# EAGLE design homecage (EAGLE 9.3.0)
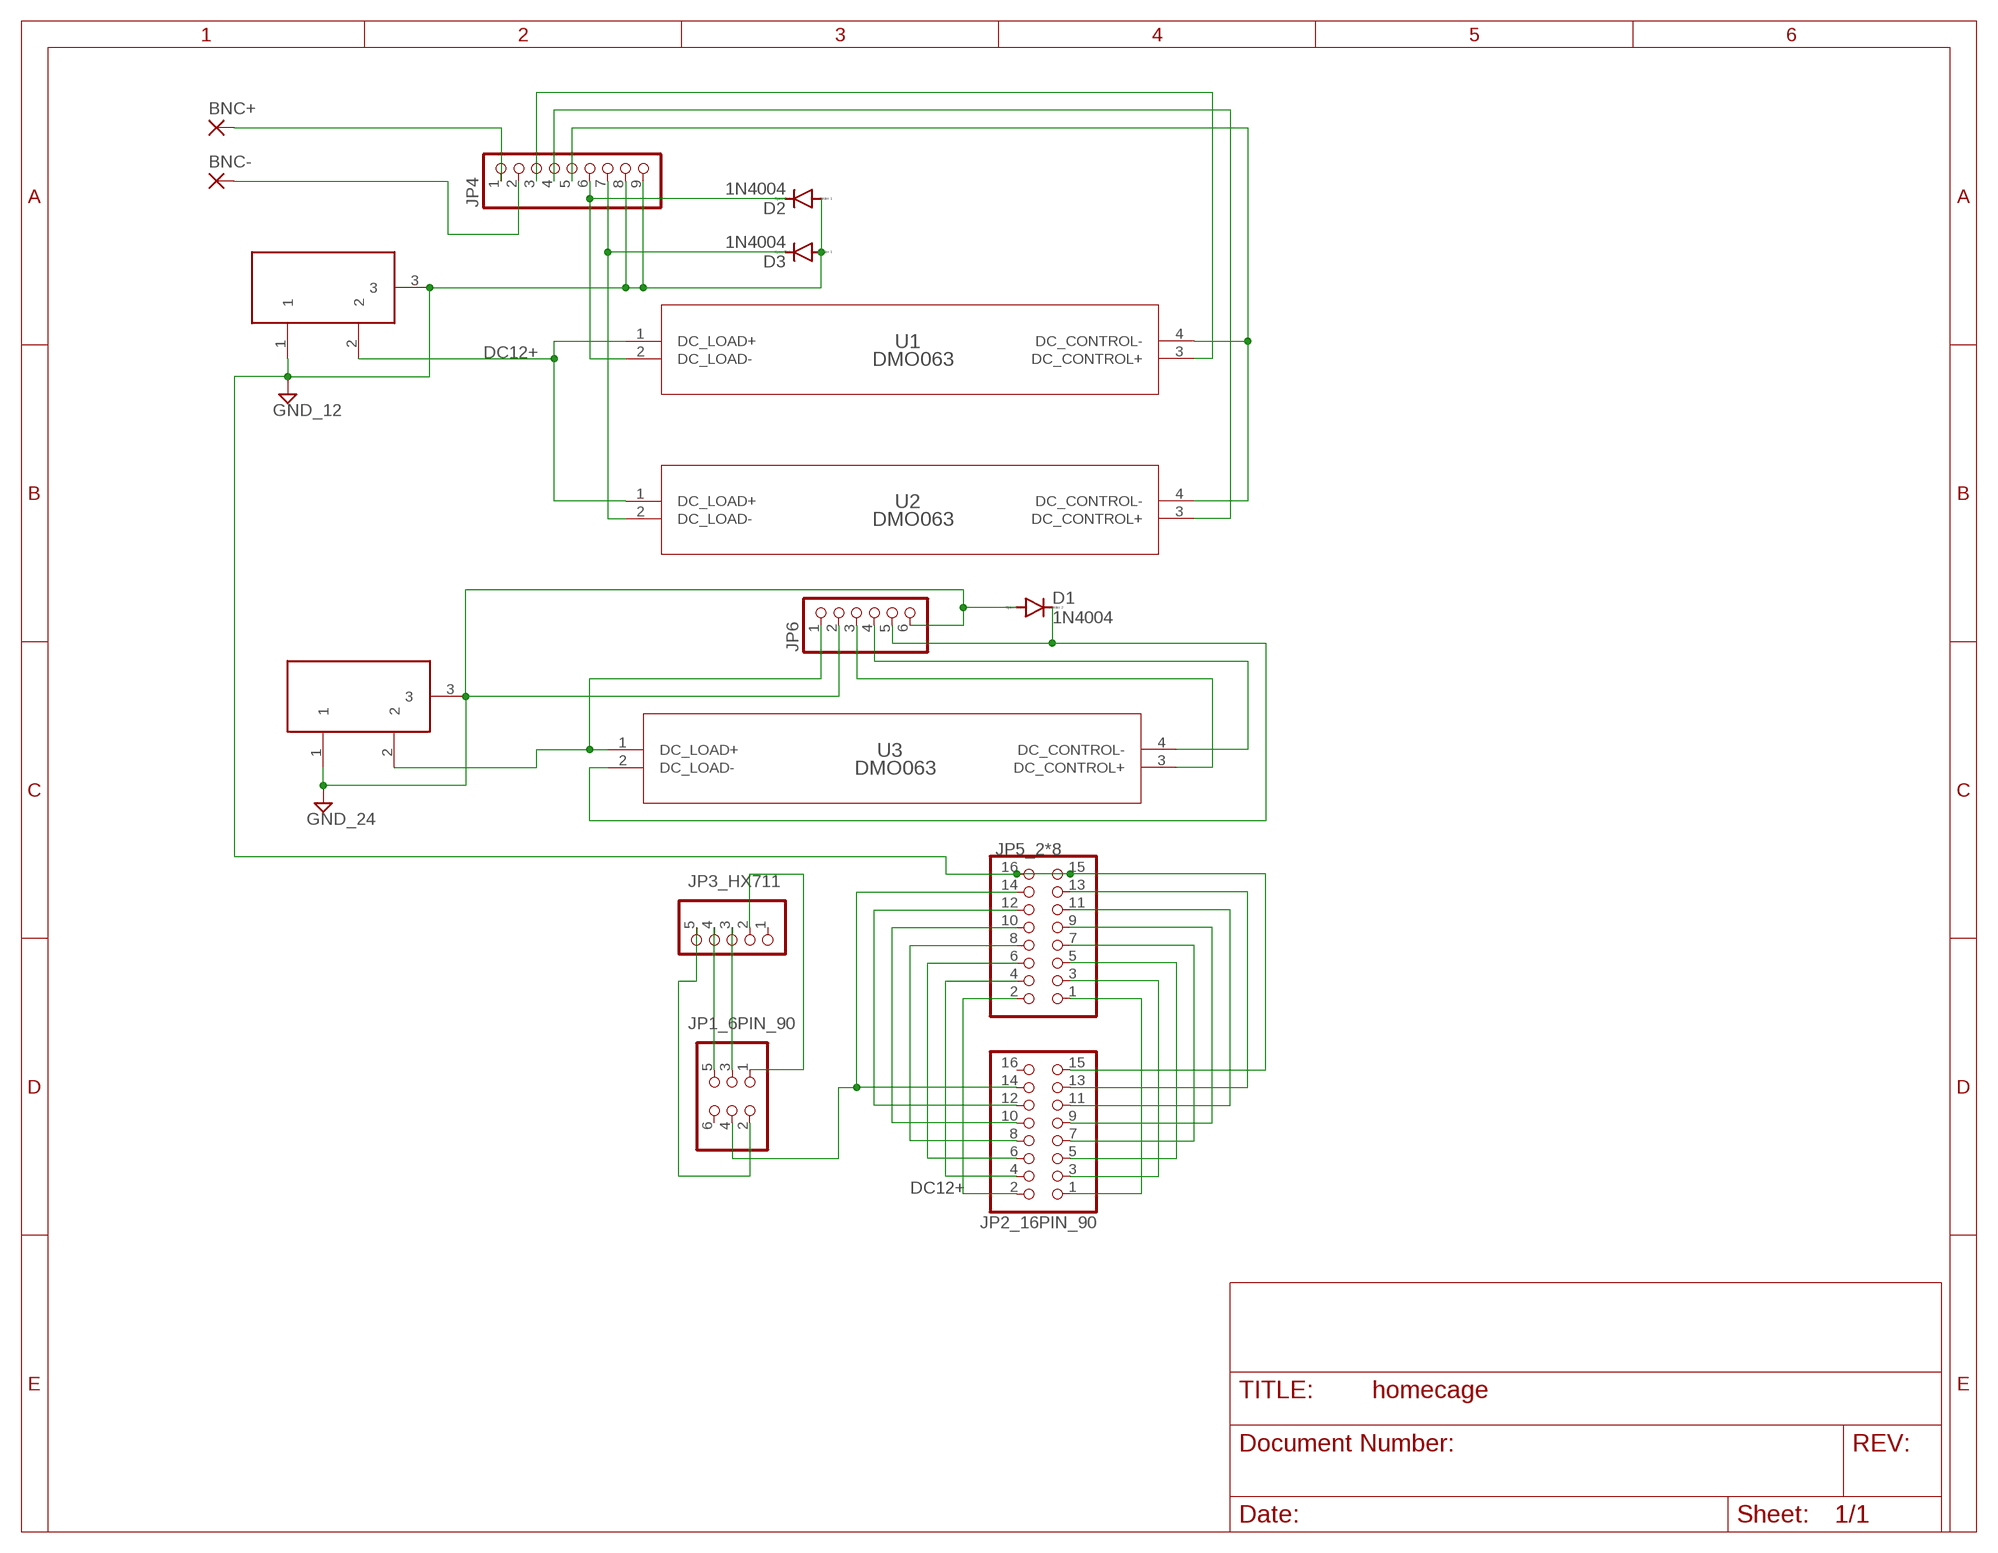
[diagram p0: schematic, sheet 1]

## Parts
BNC+  SMD5  [SMD2,54-5,08]
BNC-  SMD5  [SMD2,54-5,08]
D1  1N4004  [DO41-10]
D2  1N4004  [DO41-10]
D3  1N4004  [DO41-10]
DC12V  POWERSUPPLY_DC21MMX  [POWERSUPPLY_DC-21MM]
DC24V  POWERSUPPLY_DC21MMX  [POWERSUPPLY_DC-21MM]
JP1_6PIN_90  PINHD-2X3/90  [2X03/90]
JP2_16PIN_90  PINHD-2X8/90  [2X08/90]
JP3_HX711  PINHD-1X5  [1X05]
JP4  PINHD-1X9  [1X09]
JP5_2*8  PINHD-2X8  [2X08]
JP6  PINHD-1X6  [1X06]
U1  DMO063  [SIP-4_DMO]
U2  DMO063  [SIP-4_DMO]
U3  DMO063  [SIP-4_DMO]

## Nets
DC12+ [power]: DC12V.2 JP2_16PIN_90.2 JP5_2*8.2 U1.1(DC_LOAD+) U2.1(DC_LOAD+)
GND1 [power]: D2.A D3.A DC12V.1 DC12V.3 JP2_16PIN_90.15 JP4.8 JP4.9 JP5_2*8.15 JP5_2*8.16 ; supply symbol labelled GND_12
GND2 [power]: D1.A DC24V.1 DC24V.3 JP6.2 JP6.6 ; supply symbol labelled GND_24
N$1: JP2_16PIN_90.1 JP5_2*8.1
N$2: JP2_16PIN_90.3 JP5_2*8.3
N$3: JP2_16PIN_90.5 JP5_2*8.5
N$4: JP2_16PIN_90.7 JP5_2*8.7
N$5: JP2_16PIN_90.9 JP5_2*8.9
N$6: JP2_16PIN_90.11 JP5_2*8.11
N$7: JP2_16PIN_90.13 JP5_2*8.13
N$8: D2.C JP4.6 U1.2(DC_LOAD-)
N$10: JP2_16PIN_90.4 JP5_2*8.4
N$11: JP2_16PIN_90.6 JP5_2*8.6
N$12: JP2_16PIN_90.8 JP5_2*8.8
N$13: JP2_16PIN_90.10 JP5_2*8.10
N$14: JP2_16PIN_90.12 JP5_2*8.12
N$15: JP1_6PIN_90.4 JP2_16PIN_90.14 JP5_2*8.14
N$17: JP1_6PIN_90.1 JP3_HX711.2
N$18: JP1_6PIN_90.3 JP3_HX711.3
N$19: JP1_6PIN_90.5 JP3_HX711.4
N$20: JP1_6PIN_90.2 JP3_HX711.5
N$22 [power]: DC24V.2 JP6.1 U3.1(DC_LOAD+)
N$23: D3.C JP4.7 U2.2(DC_LOAD-)
N$24: JP4.5 U1.4(DC_CONTROL-) U2.4(DC_CONTROL-)
N$25: BNC+.1(P) JP4.1
N$26: JP4.4 U2.3(DC_CONTROL+)
N$27: JP4.3 U1.3(DC_CONTROL+)
N$28: BNC-.1(P) JP4.2
N$30: JP6.3 U3.3(DC_CONTROL+)
N$31: JP6.4 U3.4(DC_CONTROL-)
N$32: D1.C JP6.5 U3.2(DC_LOAD-)
Unconnected: JP1_6PIN_90.6 JP2_16PIN_90.16 JP3_HX711.1

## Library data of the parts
BNC+ BNC- = wirepad:SMD5: SMD PAD
D1-D3 = diode:1N4004: DIODE
DC12V DC24V = Arduino_MEGA2560_ref:POWERSUPPLY_DC21MM
JP1_6PIN_90 = pinhead:PINHD-2X3: PIN HEADER
JP2_16PIN_90 JP5_2*8 = pinhead:PINHD-2X8: PIN HEADER
JP3_HX711 = pinhead:PINHD-1X5: PIN HEADER
JP4 = pinhead:PINHD-1X9: PIN HEADER
JP6 = pinhead:PINHD-1X6: PIN HEADER
U1-U3 = homecage:DMO063; MANUFACTURER_PART_NUMBER: DMO063; VENDOR: Crydom

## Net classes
0 default: width 0.406 mm
1 power: width 1.219 mm

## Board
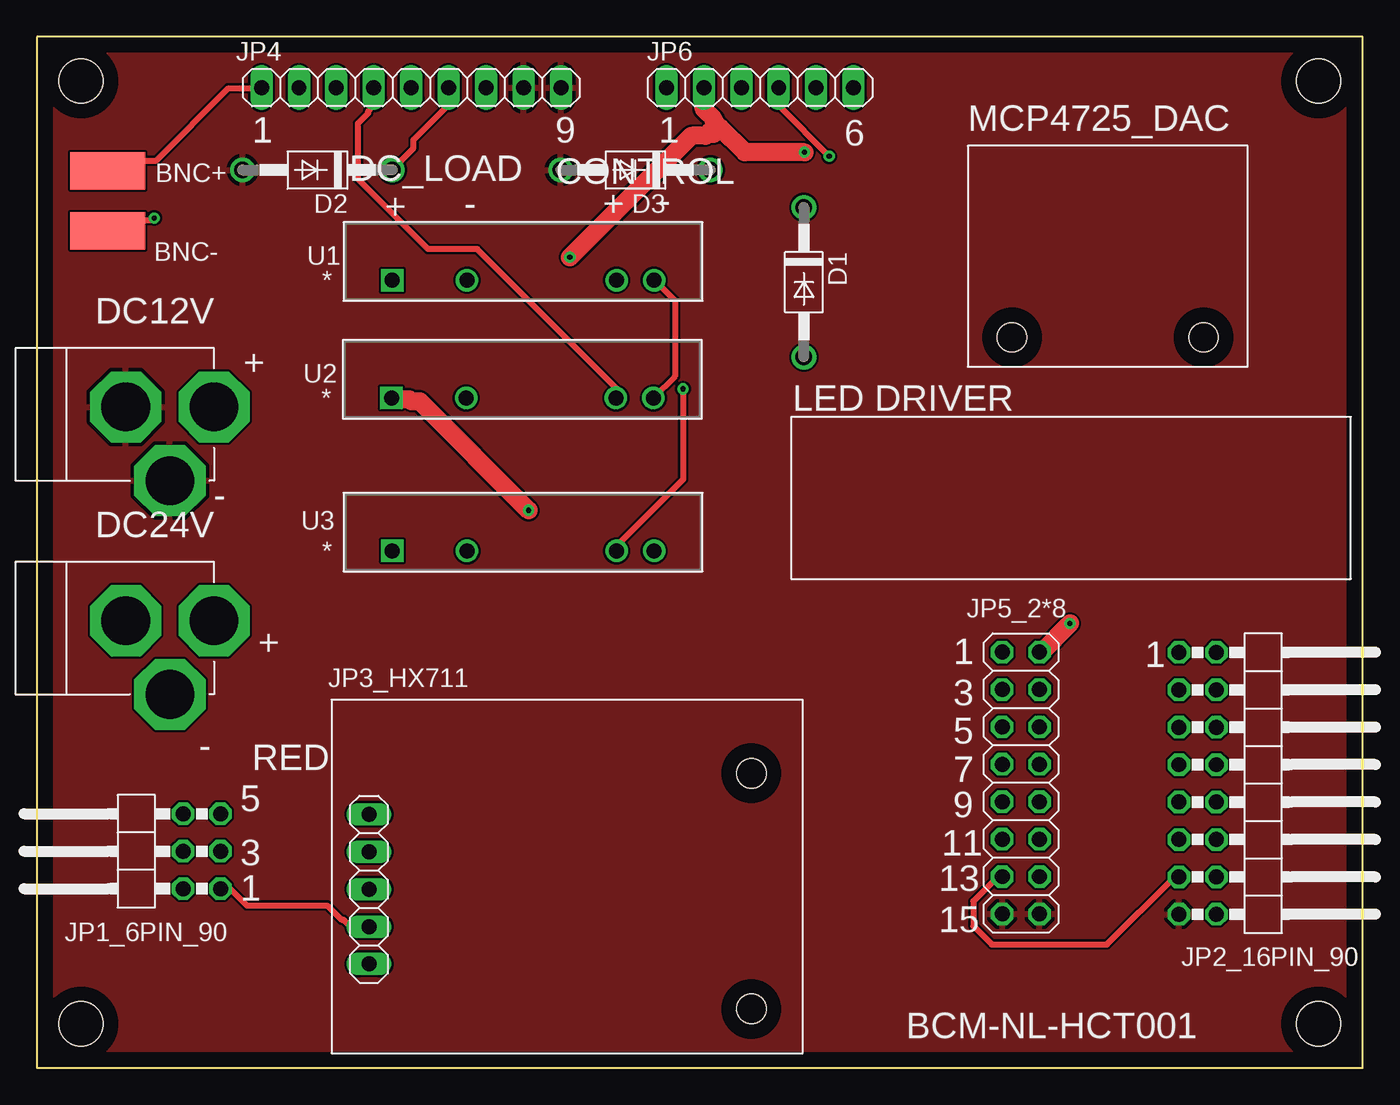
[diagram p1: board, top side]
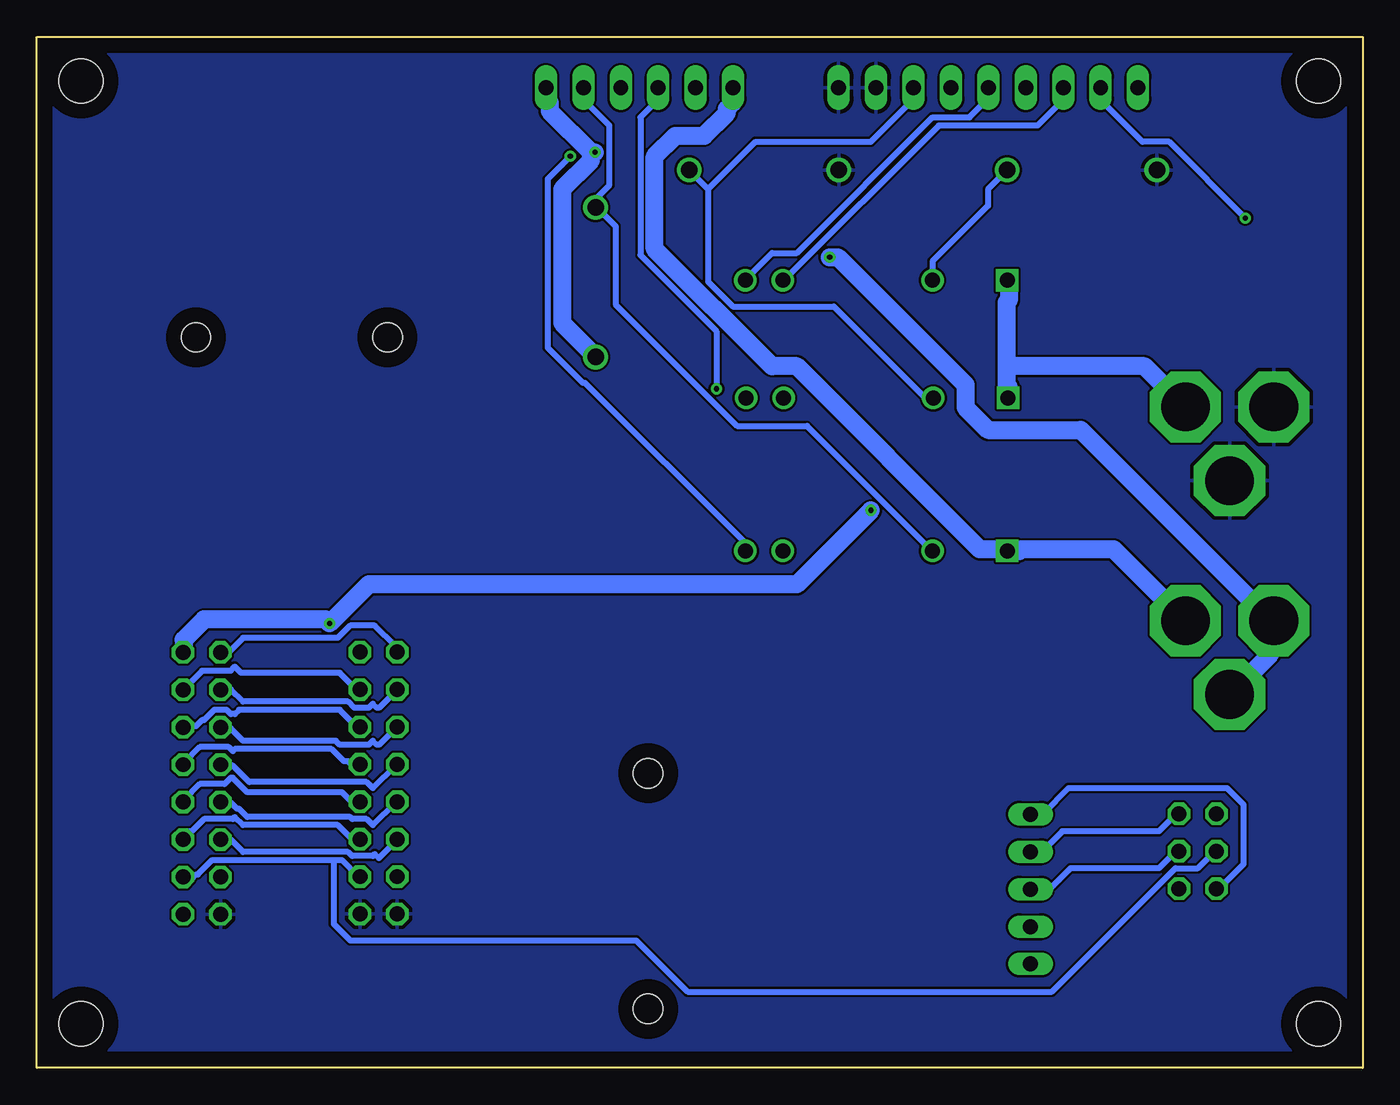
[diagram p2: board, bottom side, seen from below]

Size 90 x 70 mm. Coordinates in mm from the lower left corner, seen from the top.
Outline: 0,0 90,0 90,70 0,70 0,0
Copper layers (1*16): Top 0.035mm / dielectric 1.5mm / Bottom 0.035mm
Design rules "default": minimum track width 6mil, minimum drill 0.35mm, track to track 6mil, track to pad 6mil, pad to pad 6mil, via to via 6mil, smd to smd 6mil, copper to edge 40mil, drill to drill 6mil, minimum pad ring 10mil, minimum via ring 8mil, stop-mask expansion 4mil, vias tented up to drill 0mil, thermal gap 10mil
Holes 3 mm at 3,3 3,67 87,67 87,3
Holes 2 mm at 48.5,20 48.5,4 66.2,49.6 79.2,49.6

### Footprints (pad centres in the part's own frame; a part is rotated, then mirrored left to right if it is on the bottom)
SMD2,54-5,08 = smd 2.54 x 5.08: 1 0,0
DO41-10 = drill 1.118: A 5.08,0; C -5.08,0
POWERSUPPLY_DC-21MM = drill 3.302 pad 4.826 octagon: 1 -5.08,-3.353; 2 -0.076,-6.35; 3 -0.076,-0.356
2X03/90 = drill 1.016 octagon: 1 -2.54,-6.35; 2 -2.54,-3.81; 3 0,-6.35; 4 0,-3.81; 5 2.54,-6.35; 6 2.54,-3.81
2X08/90 = drill 1.016 octagon: 1 -8.89,-6.35; 2 -8.89,-3.81; 3 -6.35,-6.35; 4 -6.35,-3.81; 5 -3.81,-6.35; 6 -3.81,-3.81; 7 -1.27,-6.35; 8 -1.27,-3.81; 9 1.27,-6.35; 10 1.27,-3.81; 11 3.81,-6.35; 12 3.81,-3.81; 13 6.35,-6.35; 14 6.35,-3.81; 15 8.89,-6.35; 16 8.89,-3.81
1X05 = drill 1.016 long: 1 -5.08,0; 2 -2.54,0; 3 0,0; 4 2.54,0; 5 5.08,0
1X09 = drill 1.016 long: 1 -10.16,0; 2 -7.62,0; 3 -5.08,0; 4 -2.54,0; 5 0,0; 6 2.54,0; 7 5.08,0; 8 7.62,0; 9 10.16,0
2X08 = drill 1.016 octagon: 1 -8.89,-1.27; 2 -8.89,1.27; 3 -6.35,-1.27; 4 -6.35,1.27; 5 -3.81,-1.27; 6 -3.81,1.27; 7 -1.27,-1.27; 8 -1.27,1.27; 9 1.27,-1.27; 10 1.27,1.27; 11 3.81,-1.27; 12 3.81,1.27; 13 6.35,-1.27; 14 6.35,1.27; 15 8.89,-1.27; 16 8.89,1.27
1X06 = drill 1.016 long: 1 -6.35,0; 2 -3.81,0; 3 -1.27,0; 4 1.27,0; 5 3.81,0; 6 6.35,0
SIP-4_DMO = drill 1.016 pad 1.524 square: 1 -17.78,-2.54 | drill 1.016 pad 1.524: 2 -12.7,-2.54; 3 -2.54,-2.54; 4 0,-2.54

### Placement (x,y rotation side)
BNC+  4.8,60.9 90 top
BNC-  4.8,56.82 90 top
D1  52.07,53.34 270 top
D2  19.05,60.96 180 top
D3  40.64,60.96 180 top
DC12V  5.68,44.95 90 top
DC24V  5.68,30.44 90 top
JP1_6PIN_90  6.12,14.71 90 top
JP2_16PIN_90  83.88,19.32 270 top
JP3_HX711  22.55,12.13 90 top
JP4  25.41,66.55 0 top
JP5_2*8  66.8,19.34 270 top
JP6  49.09,66.55 0 top
U1  41.9,56.02 0 top
U2  41.85,48.02 0 top
U3  41.9,37.64 0 top

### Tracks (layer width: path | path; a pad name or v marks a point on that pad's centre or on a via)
DC12+  (via drill 0.35)
  Top 1.219: v70.13,30.18 68.17,28.22 JP5_2*8.2 | v33.39,37.86 25.98,45.26 25.43,45.26 25.29,45.4 24.17,45.4 U2.1
  Bottom 1.219: JP2_16PIN_90.2 80.05,28.22 80.05,29.06 78.65,30.45 70.41,30.45 v70.13,30.18 67.47,32.83 38.42,32.83 v33.39,37.86 | 24.17,47.64 24.17,51.97 24.03,52.11 24.03,53.37 U1.1 | 24.17,47.64 24.17,46.38 24.03,46.24 24.03,45.54 U2.1 | 24.17,47.64 14.81,47.64 12.15,44.98 DC12V.2
GND1
  pour Top (isolate 0.305): 0,0 0,70 90,70 90,0
  pour Bottom (isolate 0.305): 0,0 0,70 90,70 90,0
  pour Top (isolate 0.305): 0,0 0,70 90,70 90,0
  pour Top: 1.27,68.58 1.27,1.27 88.9,1.27 88.9,68.58
  pour Bottom: 1.27,68.58 1.27,1.27 88.9,1.27 88.9,68.58
GND2  (via drill 0.35)
  Top 1.219: 46.38,63.84 48.06,62.17 v52.11,62.17 | 46.38,63.84 45.96,64.26 45.96,64.4 45.26,65.1 45.26,66.5 JP6.2 | v36.18,55.04 44.42,63.28 45.4,63.28 45.68,63.56 45.82,63.42 45.96,63.42 46.38,63.84
  Bottom 1.219: DC24V.1 8.94,25.43 6.29,28.08 6.29,30.18 6.15,30.32 DC24V.3 6.57,30.73 19.14,43.31 25.43,43.31 26.96,44.84 26.96,46.38 35.62,55.04 v36.18,55.04 | 52.39,62.17 v52.11,62.17 | 52.39,62.17 55.18,64.96 55.18,65.52 55.32,65.66 55.32,66.5 JP6.6 | D1.A 52.11,48.34 54.34,50.57 54.34,59.65 52.39,61.61 52.39,62.17
N$1
  Bottom 0.406: JP2_16PIN_90.1 77.39,28.22 76.97,28.22 76,29.2 69.57,29.2 68.73,30.04 67.06,30.04 65.66,28.64 65.66,28.36 JP5_2*8.1
N$2
  Bottom 0.406: JP2_16PIN_90.3 77.39,25.7 76.83,25.7 76,24.87 68.87,24.87 68.45,24.45 67.47,24.45 67.2,24.73 66.92,24.45 66.78,24.45 65.66,25.57 JP5_2*8.3
N$3
  Bottom 0.406: JP2_16PIN_90.5 77.39,23.05 76.83,23.05 76,22.21 69.71,22.21 69.43,21.93 67.47,21.93 67.2,22.21 66.92,21.93 66.78,21.93 65.66,23.05 JP5_2*8.5
N$4
  Bottom 0.406: JP2_16PIN_90.7 77.39,20.54 76.69,20.54 75.58,19.42 67.61,19.42 67.2,19 65.66,20.54 JP5_2*8.7
N$5
  Bottom 0.406: JP2_16PIN_90.9 77.39,18.02 76.83,18.02 76.42,17.6 76.28,17.6 75.72,17.04 68.73,17.04 68.59,16.9 67.61,16.9 67.2,16.48 65.66,18.02 JP5_2*8.9
N$6
  Bottom 0.406: JP2_16PIN_90.11 77.39,15.51 76.83,15.51 76,14.67 68.87,14.67 68.59,14.39 67.2,14.39 67.06,14.53 66.78,14.25 65.52,15.51 JP5_2*8.11
N$7
  Top 0.406: JP2_16PIN_90.13 77.39,12.85 77.11,12.85 72.64,8.38 64.82,8.38 63.56,9.64 63.56,11.32 65.1,12.85 65.52,12.85 JP5_2*8.13
N$8
  Top 0.406: JP4.6 27.94,66.5 27.94,65.38 25.57,63.01 25.57,62.45 24.17,61.05 D2.C
  Bottom 0.406: U1.2 29.2,53.51 29.2,54.76 25.43,58.53 25.43,59.65 24.17,60.91 D2.C
N$10
  Bottom 0.406: JP2_16PIN_90.4 80.05,25.7 78.79,26.96 76.83,26.96 76.56,27.24 76.14,26.82 69.43,26.82 68.17,25.57 JP5_2*8.4
N$11
  Bottom 0.406: JP2_16PIN_90.6 80.05,23.19 79.21,23.19 78.79,23.61 78.65,23.61 77.95,24.31 77.11,24.31 76.83,24.03 76.56,24.03 76.28,24.31 69.43,24.31 68.17,23.05 JP5_2*8.6
N$12
  Bottom 0.406: JP2_16PIN_90.8 80.05,20.68 78.93,21.79 76.97,21.79 76.69,21.51 76.56,21.65 69.99,21.65 69.15,20.82 68.87,20.82 68.73,20.68 68.17,20.68 JP5_2*8.8
N$13
  Bottom 0.406: JP2_16PIN_90.10 80.05,18.16 78.93,19.28 77.25,19.28 76.83,19.7 76.69,19.7 75.72,18.72 69.29,18.72 68.73,18.16 68.17,18.16 JP5_2*8.10
N$14
  Bottom 0.406: JP2_16PIN_90.12 80.05,15.65 79.63,16.07 79.49,16.07 78.65,16.9 76.69,16.9 76.56,17.04 76,16.48 69.57,16.48 68.73,15.65 68.17,15.65 JP5_2*8.12
N$15
  Bottom 0.406: 69.85,14.11 78.09,14.11 79.07,13.13 79.21,13.13 79.49,12.85 80.05,12.85 JP2_16PIN_90.14 | 69.85,14.11 69.29,14.11 68.17,12.99 JP5_2*8.14 | 69.85,14.11 69.85,9.78 68.73,8.66 49.31,8.66 45.82,5.17 21.09,5.17 12.71,13.55 11.18,13.55 10.06,14.67 JP1_6PIN_90.4
N$17
  Top 0.406: JP3_HX711.2 22.49,9.64 21.23,9.64 20.82,10.06 20.68,10.06 19.7,11.04 14.25,11.04 13.13,12.15 12.57,12.15 JP1_6PIN_90.1
N$18
  Bottom 0.406: JP3_HX711.3 22.49,12.15 21.23,12.15 19.84,13.55 13.83,13.55 12.57,14.81 JP1_6PIN_90.3
N$19
  Bottom 0.406: JP3_HX711.4 22.49,14.81 21.65,14.81 20.4,16.07 13.83,16.07 12.57,17.32 JP1_6PIN_90.5
N$20
  Bottom 0.406: JP1_6PIN_90.2 9.92,12.29 9.64,12.29 8.1,13.83 8.1,17.88 9.22,19 19.98,19 21.65,17.32 22.49,17.32 JP3_HX711.5
N$22
  Bottom 1.219: DC24V.2 12.15,30.45 16.9,35.2 23.19,35.2 23.33,35.06 24.03,35.06 U3.1 24.73,35.2 25.98,35.2 38.42,47.64 40.09,47.64 48.06,55.6 48.06,61.89 46.66,63.28 44.7,63.28 43.17,64.82 43.17,65.1 42.75,65.52 42.75,66.5 JP6.1
N$23
  Bottom 0.406: 44.42,59.65 44.42,53.37 42.75,51.69 35.9,51.69 29.76,45.54 29.2,45.54 U2.2 | 44.42,59.65 45.68,60.91 D3.C | 44.42,59.65 41.21,62.87 33.39,62.87 30.59,65.66 30.59,66.5 JP4.7
N$24
  Top 0.406: U2.4 41.91,45.54 43.31,46.94 43.31,52.11 41.91,53.51 U1.4
  Bottom 0.406: JP4.5 25.43,66.5 25.43,65.8 26.68,64.54 29.2,64.54 38.42,55.32 40.09,55.32 41.91,53.51 U1.4
N$25
  Top 0.406: JP4.1 15.23,66.5 12.99,66.5 8.1,61.61 5.59,61.61 4.89,60.91 BNC+.1
N$26
  Top 0.406: JP4.4 22.77,66.5 22.77,65.24 22.49,64.96 22.49,64.82 21.79,64.12 21.79,60.35 26.54,55.6 29.9,55.6 39.4,46.1 39.4,45.54 U2.3
N$27
  Bottom 0.406: U1.3 39.26,53.51 28.78,63.98 22.07,63.98 20.4,65.66 20.4,66.5 JP4.3
N$28  (via drill 0.35)
  Top 0.406: v7.96,57.7 7.82,57.56 5.59,57.56 4.89,56.86 BNC-.1
  Bottom 0.406: v7.96,57.7 13.13,62.87 14.95,62.87 17.74,65.66 17.74,66.5 JP4.2
N$30  (via drill 0.35)
  Top 0.406: v43.87,46.1 43.87,39.95 39.4,35.48 39.4,35.2 U3.3
  Bottom 0.406: v43.87,46.1 43.87,50.01 49.03,55.18 49.03,64.54 47.92,65.66 47.92,66.5 JP6.3
N$31  (via drill 0.35)
  Top 0.406: v53.78,61.89 50.43,65.24 50.43,66.5 JP6.4
  Bottom 0.406: v53.78,61.89 55.32,60.35 55.32,48.9 52.95,46.52 52.81,46.52 41.91,35.62 41.91,35.2 U3.4
N$32
  Bottom 0.406: U3.2 29.34,35.2 37.72,43.59 42.47,43.59 50.71,51.83 50.71,57.14 51.97,58.4 D1.C 51.97,58.53 51.97,59.09 51.13,59.93 51.13,63.98 52.81,65.66 52.81,66.5 JP6.5

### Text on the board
tPlace: MCP4725_DAC | 1 | 9 | 1 | 6 | DC_LOAD | CONTROL | + | - | + | - | + | LED DRIVER | - | + | 1 | 1 | 3 | 5 | - | RED | 7 | 5 | 9 | 3 | 11 | 13 | 1 | 15 | BCM-NL-HCT001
